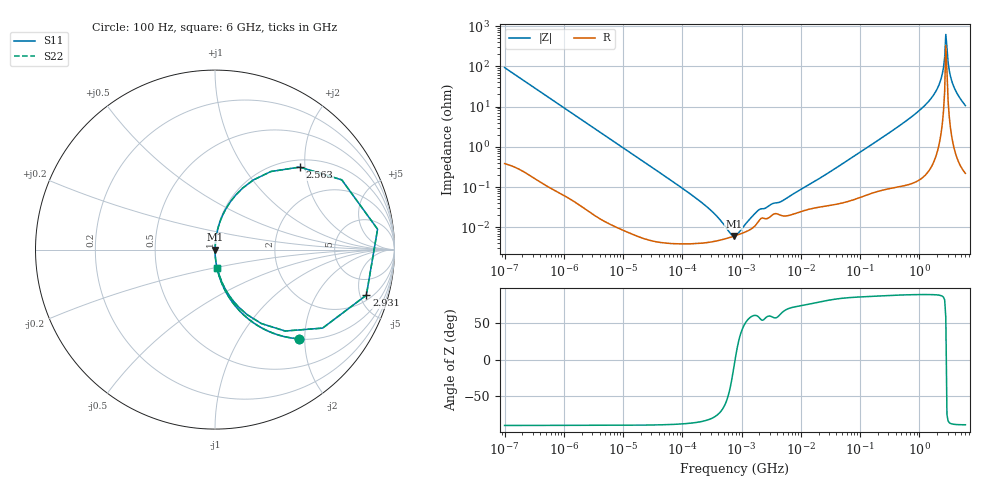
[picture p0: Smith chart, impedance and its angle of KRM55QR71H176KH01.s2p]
!Murata Part Number: KRM55QR71H176KH01
!These Parameters are Measured in Series Mode Connection
!Data Generated on Jan 08, 2026
!  o--ll--o
!Port1  Port2
!  o------o
!Operation Temp=25[degC], DC Bias Voltage=0[V]
!Freq. Start=100[Hz] Stop=6[GHz] 401[Steps]
# Hz S RI R 50
!Freq.(Hz) S11(Real) S11(Imag) S21(Real) S21(Imag) S12(Real) S12(Imag) S22(Real) S22(Imag)
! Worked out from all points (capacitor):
!   401 points, 100 Hz to 6 GHz, reference 50 ohm
!   read as one part in series: C = 17 uF near 109 Hz
!   lowest |Z| = 6.13 mohm at 740.7 kHz (marker M1)
!   series resonance near 777.4 kHz, so ESL is about 2.5 nH
!   S11 on the Smith chart (normalised r, x): 100 Hz: 1.01, -1.87; 2.563 GHz: 1.15, +1.88; 2.931 GHz: 2.52, -5.70; 6 GHz: 1.00, -0.21
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100  0.4653 -0.4967  0.5347 0.4967  0.5347 0.4967  0.4653 -0.4967
320  0.0801 -0.2686  0.9199 0.2686  0.9199 0.2686  0.0801 -0.2686
2008  0.00253 -0.0469  0.9975 0.0469  0.9975 0.0469  0.00253 -0.0469
40335  4.82e-05 -0.00235  1 0.00235  1 0.00235  4.82e-05 -0.00235
221108  4.08e-05 -0.000392  1 0.000392  1 0.000392  4.08e-05 -0.000392
541393  5.23e-05 -8.64e-05  0.9999 8.64e-05  0.9999 8.64e-05  5.23e-05 -8.64e-05
740679  6.03e-05 -1.11e-05  0.9999 1.11e-05  0.9999 1.11e-05  6.03e-05 -1.11e-05
774597  6.17e-05 -8e-07  0.9999 8e-07  0.9999 8e-07  6.17e-05 -8e-07
1059725  7.27e-05 7.07e-05  0.9999 -7.07e-05  0.9999 -7.07e-05  7.27e-05 7.07e-05
1983483  0.000148 0.000233  0.9999 -0.000233  0.9999 -0.000233  0.000148 0.000233
1.555665e7  0.000295 0.00125  0.9997 -0.00125  0.9997 -0.00125  0.000295 0.00125
3.124326e8  0.00142 0.0224  0.9986 -0.0224  0.9986 -0.0224  0.00142 0.0224
1.046602e9  0.00865 0.0838  0.9913 -0.0838  0.9913 -0.0838  0.00865 0.0838
1.873145e9  0.0547 0.2159  0.9453 -0.2159  0.9453 -0.2159  0.0547 0.2159
2.240541e9  0.1521 0.341  0.8479 -0.341  0.8479 -0.341  0.1521 0.341
2.450438e9  0.3117 0.4351  0.6883 -0.4351  0.6883 -0.4351  0.3117 0.4351
2.562649e9  0.4724 0.4598  0.5276 -0.4598  0.5276 -0.4598  0.4724 0.4598
2.802721e9  0.9058 0.1136  0.0942 -0.1136  0.0942 -0.1136  0.9058 0.1136
2.931063e9  0.8432 -0.2537  0.1568 0.2537  0.1568 0.2537  0.8432 -0.2537
3.205649e9  0.3906 -0.4536  0.6094 0.4536  0.6094 0.4536  0.3906 -0.4536
3.666503e9  0.1273 -0.3158  0.8727 0.3158  0.8727 0.3158  0.1273 -0.3158
6e9  0.0132 -0.1041  0.9868 0.1041  0.9868 0.1041  0.0132 -0.1041
